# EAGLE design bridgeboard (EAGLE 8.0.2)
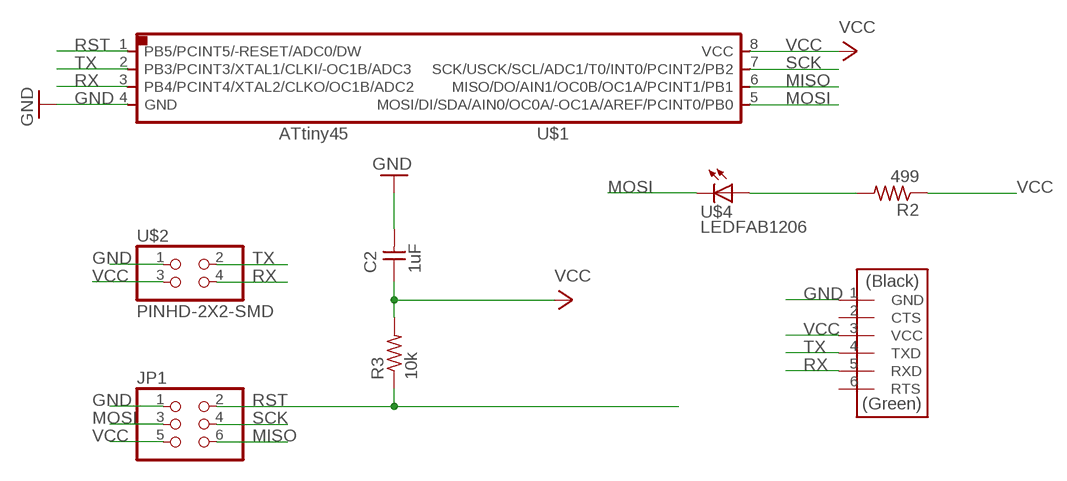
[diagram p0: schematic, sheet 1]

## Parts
C2  1uF  CAP-UNPOLARIZEDFAB  [C1206FAB]
JP1  PINHD-2X3-SMD  [2X03SMD]
R2  499  RES-US1206FAB  [R1206FAB]
R3  10k  RES-US1206FAB  [R1206FAB]
U$1  ATTINY45SI  [SOIC8]
U$2  PINHD-2X2-SMD  [2X02SMD]
U$3  FTDI-SMD-HEADER  [1X06SMD]
U$4  LEDFAB1206  [LED1206FAB]

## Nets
GND: C2.2 JP1.1 U$1.4(GND) U$2.1 U$3.1(GND)
MISO: JP1.6 U$1.6(MISO/DO/AIN1/OC0B/OC1A/PCINT1/PB1)
MOSI: JP1.3 U$1.5(MOSI/DI/SDA/AIN0/OC0A/-OC1A/AREF/PCINT0/PB0) U$4.2(C)
N$1: R2.2 U$4.1(A)
RST: JP1.2 R3.1 U$1.1(PB5/PCINT5/-RESET/ADC0/DW)
RX: U$1.3(PB4/PCINT4/XTAL2/CLKO/OC1B/ADC2) U$2.4 U$3.5(RXD)
SCK: JP1.4 U$1.7(SCK/USCK/SCL/ADC1/T0/INT0/PCINT2/PB2)
TX: U$1.2(PB3/PCINT3/XTAL1/CLKI/-OC1B/ADC3) U$2.2 U$3.4(TXD)
VCC: C2.1 JP1.5 R2.1 R3.2 U$1.8(VCC) U$2.3 U$3.3(VCC)
Unconnected: U$3.2(CTS) U$3.6(RTS)

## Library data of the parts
C2 = fab:CAP-UNPOLARIZED
JP1 = fab:PINHD-2X3-SMD: PIN HEADER
R2 R3 = fab:RES-US: Resistor (US Symbol)
U$1 = fab:ATTINY45
U$2 = fab:PINHD-2X2-SMD
U$3 = fab:FTDI-SMD-HEADER
U$4 = fab:LED: LED

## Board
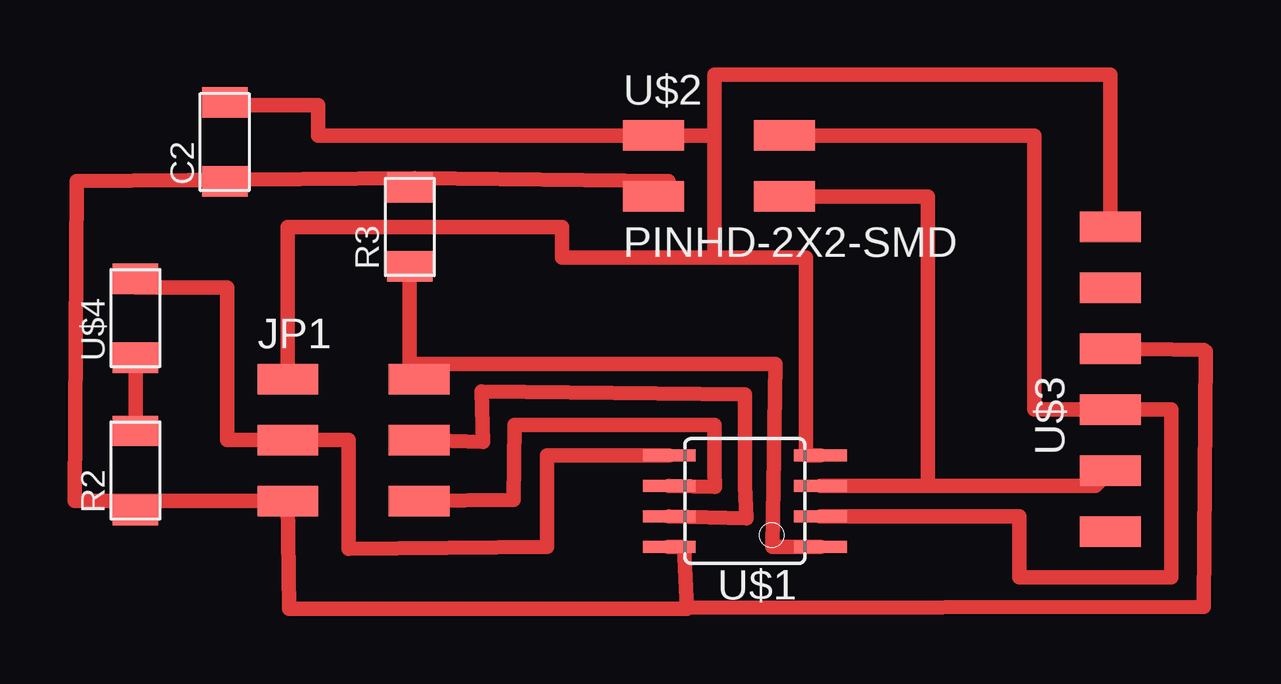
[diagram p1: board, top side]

No outline drawn. Coordinates in mm, seen from the top.
Copper layers (1*16): Top 0.035mm / dielectric 1.5mm / Bottom 0.035mm
Design rules "default *": minimum track width 24mil, minimum drill 24mil, track to track 16mil, track to pad 16mil, pad to pad 16mil, via to via 16mil, smd to smd 8mil, copper to edge 40mil, drill to drill 8mil, minimum pad ring 10mil, minimum via ring 8mil, stop-mask expansion 4mil, vias tented up to drill 0mil, thermal gap 10mil

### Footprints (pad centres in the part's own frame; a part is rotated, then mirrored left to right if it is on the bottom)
C1206FAB = smd 1.27 x 1.905: 1 -1.651,0; 2 1.651,0
2X03SMD = smd 2.54 x 1.27: 1 -2.54,2.54; 2 2.92,2.54; 3 -2.54,0; 4 2.92,0; 5 -2.54,-2.54; 6 2.92,-2.54
R1206FAB = smd 1.27 x 1.905: 1 -1.651,0; 2 1.651,0
SOIC8 = smd 0.5 x 2.2: 1 -1.905,-3.154; 2 -0.645,-3.154; 3 0.625,-3.154; 4 1.895,-3.154; 5 1.905,3.154; 6 0.635,3.154; 7 -0.635,3.154; 8 -1.905,3.154
2X02SMD = smd 2.54 x 1.27: 1 -2.54,1.27; 2 2.92,1.27; 3 -2.54,-1.27; 4 2.92,-1.27
1X06SMD = smd 2.54 x 1.27: 1 0,6.35; 2 0,3.81; 3 0,1.27; 4 0,-1.27; 5 0,-3.81; 6 0,-6.35
LED1206FAB = smd 1.27 x 1.905: 1 -1.651,0; 2 1.651,0

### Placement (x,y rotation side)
C2  -24.22,1 90 top
JP1  -19.05,-11.43 0 top
R2  -27.94,-12.7 90 top
R3  -16.51,-2.54 90 top
U$1  -2.54,-13.97 90 top
U$2  -3.81,0 0 top
U$3  12.7,-8.89 0 top
U$4  -27.94,-6.35 90 top

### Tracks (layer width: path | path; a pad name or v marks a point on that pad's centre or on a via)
GND
  Top 0.61: -3.81,-3.81 -3.81,1.27 | -3.81,1.27 U$2.1 -20.32,1.27 -20.32,2.54 -24.13,2.54 C2.2 | U$1.4 0,-12.06 0,-3.81 -3.81,-3.81 | JP1.1 -21.59,-2.54 -10.16,-2.54 -10.16,-3.81 -3.81,-3.81 | -3.81,1.27 -3.81,3.81 12.7,3.81 U$3.1
MISO
  Top 0.61: U$1.6 -3.79,-13.38 -3.81,-12.7 -3.81,-10.79 -12.15,-10.79 -12.18,-13.93 JP1.6
MOSI
  Top 0.61: U$4.2 -27.94,-5.08 -24.13,-5.08 -24.13,-11.43 JP1.3 -19.05,-11.43 -19.05,-13.97 -19.07,-15.96 -10.79,-15.88 -10.79,-12.06 U$1.5
N$1
  Top 0.61: U$4.1 R2.2
RST
  Top 0.61: -16.51,-8.26 -16.51,-8.89 JP1.2 | -16.51,-8.26 R3.1 | U$1.1 -0.64,-15.88 -1.4,-15.89 -1.27,-8.26 -16.51,-8.26
RX
  Top 0.61: 5.08,-13.34 12.06,-13.34 U$3.5 | 5.08,-13.34 0.64,-13.34 U$1.3 | 5.08,-13.34 5.08,-1.27 U$2.4
SCK
  Top 0.61: U$1.7 -2.46,-14.69 -2.54,-13.34 -2.54,-9.53 -13.51,-9.39 -13.46,-11.52 JP1.4
TX
  Top 0.61: U$1.2 0.64,-14.61 8.89,-14.61 8.89,-17.14 15.24,-17.14 15.24,-10.16 U$3.4 9.53,-10.16 9.53,1.27 U$2.2
VCC
  Top 0.61: -25.73,-0.59 -30.39,-0.64 -30.48,-13.97 -27.94,-13.97 | -25.73,-0.59 -16.34,-0.51 | U$2.3 -5.71,-0.64 -16.34,-0.51 | -16.34,-0.51 R3.2 | -27.94,-13.97 JP1.5 -21.55,-18.47 -4.95,-18.47 | -5.71,-15.88 U$1.8 -5.08,-15.88 -4.95,-18.47 | U$3.3 16.58,-7.67 16.68,-7.73 16.59,-18.38 -5.08,-18.41 -4.95,-18.47 | -27.94,-13.97 R2.1 | C2.1 -24.22,-0.59 -25.73,-0.59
